(* Logix 5000 Program export EMULATE_TCP_SOCKET; software revision 36.00 *)

TYPE DATATYPE_EMULATION_SOCKET :   // Datatype of FACTORY_IO_SOCKET
STRUCT
   STATUS_CODE : DINT;   // Status code of the socket operation
   CONFIG_SERVER_PORT : STRING_0005;   // Server port number
   CONFIG_SERVER_IP : STRING_0015;   // Server IP address
   CONFIG_MODULE_PATH : STRING;   // Ethernet card path input
   CONFIG_TIMEOUT : DINT;   // Timeout input
   CONFIG_LINGER : DINT;   // Linger input
   CONFIG_QUEUE_SIZE : DINT;
   PARAMS_CREATE_INSTANCE : DINT;   // Instance input
   PARAMS_CREATE : DATATYPE_EMULATION_SOCKET_CREATE;   // Parameters for socket creation
   PARAMS_OPEN : DATATYPE_EMULATION_SOCKET_OPEN;   // Parameters for opening socket
   PARAMS_OPEN_REQUIRED_LENGTH : DINT;
   PARAMS_READ : DATATYPE_EMULATION_SOCKET_READ;   // Parameters for reading from socket
   PARAMS_READ_DESTINATION : DATATYPE_EMULATION_SOCKET_READ_DEST;   // Socket response data
   PARAMS_WRITE : DATATYPE_EMULATION_SOCKET_WRITE;   // Parameters for writing to socket
   PARAMS_WRITE_SIZE_SENT : DINT;   // Size of data sent during write operation
   INPUT_ENABLE_SOCKET : BOOL;   // Enable socket operation
   INPUT_RESET : BOOL;
   READ_LATCH : BOOL;
   READ_QUEUE : STRING_0256[250];
   READ_STRING_ENQUEUE : STRING_0256;
   READ_STRING_ENQUEUE_BUFFER : STRING_3984;
   READ_STRING_ENQUEUE_BUFFER_OLD : STRING_3984;
   READ_STRING_DEQUEUE : STRING_0256;
   READ_TAIL : DINT;
   READ_COUNT : DINT;
   READ_HEAD : DINT;
   WRITE_LATCH : BOOL;
   WRITE_QUEUE : STRING_0256[250];
   WRITE_STRING_ENQUEUE : STRING_0256;
   WRITE_STRING_DEQUEUE : STRING_0256;
   WRITE_HEAD : DINT;
   WRITE_COUNT : DINT;
   WRITE_TAIL : DINT;
   DUMMY_DINT_READ : DINT[5];
   DUMMY_DINT_WRITE : DINT[5];
END_STRUCT
END_TYPE

TYPE DATATYPE_EMULATION_SOCKET_ADDRESS :   // Datatype of FACTORY_IO_SOCKET_ADDRESS
STRUCT
   Family : INT;   // Address Family Must be 2
   Port : INT;   // Port Number
   Addr : SINT[4];   // IP Address
END_STRUCT
END_TYPE

TYPE DATATYPE_EMULATION_SOCKET_CREATE :   // Datatype of FACTORY_IO_SOCKET_CREATE
STRUCT
   Type : DINT;   // 1 - TCP 2- UPD
   Addr : DATATYPE_EMULATION_SOCKET_ADDRESS;   // Socket address information
END_STRUCT
END_TYPE

TYPE DATATYPE_EMULATION_SOCKET_OPEN :   // Datatype of FACTORY_IO_SOCKET_OPEN
STRUCT
   Timeout : DINT;   // Timeout for opening socket
   DestAddr : STRING;   // Destination address
END_STRUCT
END_TYPE

TYPE DATATYPE_EMULATION_SOCKET_READ :   // Datatype of FACTORY_IO_SOCKET_READ
STRUCT
   Timeout : DINT;   // Timeout for reading from socket
   BufLen : DINT;   // Buffer length for read operation
END_STRUCT
END_TYPE

TYPE DATATYPE_EMULATION_SOCKET_READ_DEST :   // Datatype of FACTORY_IO_SOCKET_RESPONSE
STRUCT
   FromAddr : DATATYPE_EMULATION_SOCKET_ADDRESS;   // Source address of the response
   Buffer : STRING_3984;   // Response buffer
END_STRUCT
END_TYPE

TYPE DATATYPE_EMULATION_SOCKET_WRITE :   // Datatype of FACTORY_IO_SOCKET_WRITE
STRUCT
   Timeout : DINT;   // Timeout for writing to socket
   ToAddr : DATATYPE_EMULATION_SOCKET_ADDRESS;   // Destination address for write operation
   Buffer : STRING_3972;   // Write buffer
END_STRUCT
END_TYPE

TYPE STRING_0005 :   // string type
STRUCT
   LEN : DINT;
   DATA : SINT[5];
END_STRUCT
END_TYPE

TYPE STRING_0015 :   // string type
STRUCT
   LEN : DINT;
   DATA : SINT[15];
END_STRUCT
END_TYPE

TYPE STRING_0256 :   // string type
STRUCT
   LEN : DINT;
   DATA : SINT[256];
END_STRUCT
END_TYPE

TYPE STRING_3972 :   // string type
STRUCT
   LEN : DINT;
   DATA : SINT[3972];
END_STRUCT
END_TYPE

TYPE STRING_3984 :   // string type
STRUCT
   LEN : DINT;
   DATA : SINT[3984];
END_STRUCT
END_TYPE

ADD_ON_INSTRUCTION AOI_EMULATION_SOCKET   (* revision 1.0 *)
// AOI to communicate with factory IO
VAR_IN_OUT
   DT_Socket : DATATYPE_EMULATION_SOCKET; {required}   // This tags holds all the data used by the messages
   MSG_Create : MESSAGE; {required}   // Create socket
   MSG_Open : MESSAGE; {required}   // Connect socket to server.
   MSG_Read : MESSAGE; {required}   // Message to tell socket to return any data it has recieved
   MSG_Write : MESSAGE; {required}   // Write socket message
   MSG_Delete : MESSAGE; {required}   // Delete socket
   MSG_Linger : MESSAGE; {required}   // Linger Featuer Message
END_VAR
VAR_OUTPUT
   status_enable : BOOL; {access None, visible}
   status_creating_socket : BOOL; {access None, visible}
   status_connecting : BOOL; {access None, visible}
   status_open : BOOL; {access None, visible}
   status_read : BOOL; {access None, visible}
   status_write : BOOL; {access None, visible}
   status_error : BOOL; {access None, visible}
   status_reading : BOOL; {access None, visible}
   status_writing : BOOL; {access None, visible}
   socket_state : DINT; {access None, visible}
END_VAR
VAR_INPUT
   test_reset_ons : BOOL; {access None, visible}
END_VAR
VAR_OUTPUT
   status_read_queue_not_full : BOOL; {access None, visible}
   max_enque_index : DINT; {access None, visible}
END_VAR
VAR
   State : DINT := 60;   // Current state
   temp : STRING; {access None}
   ons_reset : BOOL; {access None}
   path_string : STRING; {access None}
   read_head : DINT; {access None}
   read_count : DINT; {access None}
   const_port_config : STRING_0015; {access None}
   temp_start_pos : DINT; {access None}
   temp_total_lenght : DINT; {access None}
   temp_index : DINT; {access None}
   const_CRLF : STRING; {access None}
   temp_crlfpos : DINT; {access None}
   temp_string_to_queue : STRING_3984; {access None}
END_VAR

ROUTINE Logic   (* structured text *)
   
   
   if s:fs or (DT_Socket.INPUT_RESET and ons_reset) or test_reset_ons then
   //if  test_reset_ons then ns then
   
   	DT_Socket.CONFIG_QUEUE_SIZE := 200;
   	DT_Socket.READ_HEAD  := 0;
   	DT_Socket.READ_TAIL  := 0;
   	DT_Socket.READ_COUNT := 0;
   	DT_Socket.WRITE_HEAD  := 0;
   	DT_Socket.WRITE_TAIL  := 0;
   	DT_Socket.WRITE_COUNT := 0;
   
   	test_reset_ons := 0;
   	const_port_config := '?PORT=';
   	const_CRLF := '$r$l';
   	max_enque_index := 0;
   
   	path_string := '';
   	CONCAT(path_string, DT_Socket.CONFIG_SERVER_IP, path_string);
   	CONCAT(path_string, const_port_config , path_string);
   	CONCAT(path_string, DT_Socket.CONFIG_SERVER_PORT, path_string);
   	DT_Socket.PARAMS_OPEN.DestAddr := path_string;
   
   	MSG_Create.Path := DT_Socket.CONFIG_MODULE_PATH;
   	MSG_Open.Path 	:= DT_Socket.CONFIG_MODULE_PATH;
   	MSG_Read.Path 	:= DT_Socket.CONFIG_MODULE_PATH;
   	MSG_Write.Path 	:= DT_Socket.CONFIG_MODULE_PATH;
   	MSG_Delete.Path := DT_Socket.CONFIG_MODULE_PATH;
   	MSG_Linger.Path := DT_Socket.CONFIG_MODULE_PATH;
   
   	DT_Socket.PARAMS_OPEN.Timeout 	:= DT_Socket.CONFIG_TIMEOUT;
   	DT_Socket.PARAMS_READ.Timeout 	:= DT_Socket.CONFIG_TIMEOUT;
   	DT_Socket.PARAMS_WRITE.Timeout 	:= DT_Socket.CONFIG_TIMEOUT;
   
   	status_enable			:= 0;
   	status_creating_socket	:= 0;
   	status_connecting		:= 0;
   	status_open				:= 0;
   	status_read				:= 0;
   	status_reading				:= 0;
   	status_write			:= 0;
   	status_writing			:= 0;
   	status_error			:= 0;
   	socket_state := 0;
   
   end_if;
   ons_reset := not DT_Socket.INPUT_RESET;
   
   
   // --- STATE MACHINE FOR TCP CLIENT ---
   CASE socket_state OF
       0: // IDLE / RESET
           socket_state := 10;
       10: // CREATE SOCKET
           //msg_Create.RemoteElement := "";
   		if not MSG_Create.EN then
   			MSG_Create.DN := 0;
   			MSG_Create.ER := 0;
   			MSG(MSG_Create);
   		end_if;
   
           IF MSG_Create.DN THEN
   			MSG_Create.EN := 0;
   			socket_state := 20;
   		end_if;
           IF MSG_Create.ER THEN
   			MSG_Create.EN := 0;
   			socket_state := 100;
   		end_if; // Error
   
   	20: // Lingering
   		MSG_Linger.Instance := DT_Socket.PARAMS_CREATE_INSTANCE;
   		if not MSG_Linger.EN then
   			MSG_Linger.DN := 0;
   			MSG_Linger.ER := 0;
   			MSG(MSG_Linger);
   		end_if;
           IF MSG_Linger.DN THEN
   			MSG_Linger.EN := 0;
   			socket_state := 30;
   		end_if;
           IF MSG_Linger.ER THEN
   			MSG_Linger.EN := 0;
   			socket_state := 100;
   		end_if;
   
       30: // CONNECT TO SERVER
           // Set MyAddress.Addr (Hex), MyAddress.Port, and MyAddress.Family (2)
           MSG_Open.Instance := DT_Socket.PARAMS_CREATE_INSTANCE;
   		MSG_Open.REQ_LEN := DT_Socket.PARAMS_OPEN_REQUIRED_LENGTH;
           if not MSG_Open.EN then
   			MSG_Open.DN := 0;
   			MSG_Open.ER := 0;
   
   			MSG(MSG_Open);
   		end_if;
   
           IF MSG_Open.DN THEN
   			MSG_Open.EN := 0;
   
   			MSG_Read.Instance  := DT_Socket.PARAMS_CREATE_INSTANCE;
   			MSG_Write.Instance := DT_Socket.PARAMS_CREATE_INSTANCE;
   			socket_state := 40;
   		end_if;
           IF MSG_Open.ER THEN
   			MSG_Open.EN := 0;
   			socket_state := 100;
   		end_if;
   
   	40:
   		// Read Logic
   		if not MSG_Read.EN then
   			MSG_Read.DN := 0;
   			MSG_Read.ER := 0;
   			MSG(MSG_Read);
   		end_if;
   
   		if MSG_Read.DN   then
   			MSG_Read.EN := 0;
   			if DT_Socket.PARAMS_READ_DESTINATION.Buffer.LEN > 0 then
   				CONCAT(DT_Socket.READ_STRING_ENQUEUE_BUFFER, DT_Socket.PARAMS_READ_DESTINATION.Buffer, DT_Socket.READ_STRING_ENQUEUE_BUFFER);
   				// here can be added old data not proceeded
   				 DT_Socket.PARAMS_READ_DESTINATION.Buffer.LEN := 0;
   			end_if;
   		end_if;
   
   		IF MSG_Read.ER THEN
   			MSG_Read.EN := 0;
   			socket_state := 100;
   		end_if;
   
   		// Write Logic
   		if DT_Socket.WRITE_LATCH then
   			DT_Socket.WRITE_LATCH := 0;
   			MSG_Write.DN := 0;
   			MSG_Write.ER := 0;
   			COP(DT_Socket.WRITE_STRING_DEQUEUE,DT_Socket.PARAMS_WRITE.Buffer,1);
   			MSG_Write.REQ_LEN := DT_Socket.PARAMS_WRITE.Buffer.LEN + 16;
   			MSG(MSG_Write);
   
   			/*
   			if not MSG_Write.EN  then
   				MSG_Write.DN := 0;
   				MSG_Write.ER := 0;
   
   				COP(DT_Socket.WRITE_STRING_DEQUEUE,DT_Socket.Params_Write.Buffer,1);
   				MSG_Write.REQ_LEN := DT_Socket.Params_Write.Buffer.LEN + 16;
   				MSG(MSG_Write);
   			end_if;
   			*/
   		end_if;
   
   		if MSG_Write.DN  then
   			MSG_Write.EN := 0;
   			MSG_Write.DN := 0;
   			DT_Socket.PARAMS_WRITE.Buffer := '';
   		end_if;
   
   		if MSG_Write.ER then
   			MSG_Write.EN := 0;
   			MSG_Write.ER := 0;
   			socket_state := 100;
   		end_if;
   
       100: // DELETE SOCKET (CLEANUP ON ERROR OR CLOSE)
           MSG_Delete.Instance := DT_Socket.PARAMS_CREATE_INSTANCE;
   		if not MSG_Delete.EN then
   			MSG_Delete.DN := 0;
   			MSG_Delete.ER := 0;
           	MSG(MSG_Delete);
   		end_if;
   
           IF MSG_Delete.DN or MSG_Delete.ER then
   			MSG_Delete.EN := 0;
   			socket_state := 0;
   			//test_reset_ons := 1;
   		end_if;
   END_CASE;
   
   
   //////////////////////////////
   // Write Deque
   IF not DT_Socket.WRITE_LATCH AND MSG_Open.DN and (DT_Socket.WRITE_COUNT > 0) THEN
       CPS(DT_Socket.WRITE_QUEUE[DT_Socket.WRITE_HEAD], DT_Socket.WRITE_STRING_DEQUEUE, 1);
       DT_Socket.WRITE_HEAD := (DT_Socket.WRITE_HEAD + 1) MOD DT_Socket.CONFIG_QUEUE_SIZE;
       DT_Socket.WRITE_COUNT := DT_Socket.WRITE_COUNT - 1;
   	DT_Socket.WRITE_LATCH := 1;
   END_IF;
   
   
   /////////////////////////////
   // Read Enque
   
   temp_start_pos := 1;
   temp_total_lenght := 0;
   temp_crlfpos := 1;
   
   if DT_Socket.READ_STRING_ENQUEUE_BUFFER.LEN > 0 then
   	for temp_index := 0 to 20 do
   
   		if temp_index > max_enque_index then
   			max_enque_index := temp_index ;
   		end_if;
   
   		IF temp_start_pos >= DT_Socket.READ_STRING_ENQUEUE_BUFFER.LEN THEN EXIT; END_IF;
   		FIND(DT_Socket.READ_STRING_ENQUEUE_BUFFER, const_CRLF, temp_start_pos, temp_crlfpos);
   
   		temp_total_lenght := temp_crlfpos - temp_start_pos;
   		 MID(DT_Socket.READ_STRING_ENQUEUE_BUFFER, temp_total_lenght, temp_start_pos, temp_string_to_queue);
   		status_read_queue_not_full := DT_Socket.READ_COUNT < DT_Socket.CONFIG_QUEUE_SIZE;
   
   		IF status_read_queue_not_full THEN
   			CONCAT(temp_string_to_queue, const_CRLF, temp_string_to_queue);
   			CPS( temp_string_to_queue, DT_Socket.READ_QUEUE[DT_Socket.READ_TAIL], 1);
       		DT_Socket.READ_TAIL := (DT_Socket.READ_TAIL + 1) MOD DT_Socket.CONFIG_QUEUE_SIZE;
       		DT_Socket.READ_COUNT := DT_Socket.READ_COUNT + 1;
   		END_IF;
   
   
   		temp_start_pos := temp_crlfpos +2;
   	end_for;
   
   
   
   	DT_Socket.READ_STRING_ENQUEUE_BUFFER := '';
   end_if;
   
   
   /*
   //////////////////////////////
   // Read Deque
   IF not DT_Socket.WRITE_LATCH AND MSG_Open.DN and (read_count > 0) THEN
       CPS(DT_Socket.READ_QUEUE[write_head], DT_Socket.READ_STRING_DEQUEUE, 1);
       read_head := (read_head + 1) MOD DT_Socket.CONFIG_QUEUE_SIZE;
       read_count := read_count - 1;
   	DT_Socket.WRITE_LATCH := 1;
   END_IF;
   */
   
   
   
   
   // HMI
   
   
END_ROUTINE
END_ADD_ON_INSTRUCTION

ADD_ON_INSTRUCTION AOI_EMULATION_SOCKET_DEQUEUE_READ   (* revision 1.0 *)
VAR_IN_OUT
   DT_Socket : DATATYPE_EMULATION_SOCKET; {required}   // This tags holds all the data used by the messages
END_VAR
VAR_OUTPUT
   status_new_messages : BOOL; {access None, visible}
   status_empty : DINT; {access None}
END_VAR
VAR_INPUT
   reset_stats_ons : BOOL; {access None, visible}
END_VAR
VAR_OUTPUT
   counts_good : DINT; {access None, visible}
   counts_bad : DINT; {access None, visible}
END_VAR
VAR
   ons_reset : BOOL; {access None}
   sCrLf : STRING; {access None}
   last_message : STRING_0256; {access None}
   size_message : DINT; {access None}
END_VAR

ROUTINE Logic   (* structured text *)
   
   /* //delete if not used
   
   if s:fs or (DT_Socket.INPUT_RESET and ons_reset)  then
   	DT_Socket.CONFIG_QUEUE_SIZE := 200;
   end_if;
   ons_reset := not DT_Socket.INPUT_RESET;
   */
   
   if reset_stats_ons then
   	reset_stats_ons:= 0;
   	counts_good:= 0;
   	counts_bad:= 0;
   end_if;
   
   status_new_messages := DT_Socket.READ_COUNT > 0;
   
   IF status_new_messages THEN
       CPS(DT_Socket.READ_QUEUE[DT_Socket.READ_HEAD], last_message, 1);
       DT_Socket.READ_HEAD := (DT_Socket.READ_HEAD + 1) MOD DT_Socket.CONFIG_QUEUE_SIZE;
       DT_Socket.READ_COUNT := DT_Socket.READ_COUNT - 1;
   	DT_Socket.READ_LATCH := 1;
   END_IF;
   
   
   // Parse Message
   size_message := 200;
   
   //if (DT_Socket.READ_LATCH and (last_message.DATA[size_message - 2] = 13) and (last_message.DATA[size_message - 1] = 10)) then
   if (last_message.LEN = size_message) then
   	CPS(last_message,DT_Socket.READ_STRING_DEQUEUE, 1);
   
   	counts_good := counts_good +1;
   else
   	counts_bad := counts_bad +1;
   end_if;
   
   
   
   
   
   
   
   
   
END_ROUTINE
END_ADD_ON_INSTRUCTION

ADD_ON_INSTRUCTION AOI_EMULATION_SOCKET_ENQUEUE_SEND   (* revision 1.0 *)
VAR_IN_OUT
   DT_Socket : DATATYPE_EMULATION_SOCKET; {required}   // This tags holds all the data used by the messages
END_VAR
VAR_OUTPUT
   status_full : BOOL; {access None, visible}
   status_empty : DINT; {access None}
END_VAR
VAR
   ons_reset : BOOL; {access None}
   sCrLf : STRING; {access None}
   const_CRLF : STRING; {access None}
   fix_lenght : DINT; {access None}
END_VAR

ROUTINE Logic   (* structured text *)
   
   /* // delete if not used
   if s:fs or (DT_Socket.INPUT_RESET and ons_reset)  then
   	DT_Socket.CONFIG_QUEUE_SIZE := 200;
   end_if;
   ons_reset := not DT_Socket.INPUT_RESET;
   */
   DT_Socket.WRITE_STRING_ENQUEUE.LEN := 198;
   const_CRLF := '$r$l';
   status_full := DT_Socket.WRITE_COUNT > DT_Socket.CONFIG_QUEUE_SIZE;
   
   IF not status_full THEN
   	CONCAT(DT_Socket.WRITE_STRING_ENQUEUE, const_CRLF, DT_Socket.WRITE_STRING_ENQUEUE);
   	CPS( DT_Socket.WRITE_STRING_ENQUEUE, DT_Socket.WRITE_QUEUE[DT_Socket.WRITE_TAIL], 1);
       DT_Socket.WRITE_TAIL := (DT_Socket.WRITE_TAIL + 1) MOD DT_Socket.CONFIG_QUEUE_SIZE;
       DT_Socket.WRITE_COUNT := DT_Socket.WRITE_COUNT + 1;
   END_IF;
   
   
   
   
   
END_ROUTINE
END_ADD_ON_INSTRUCTION

VAR_GLOBAL   (* controller tags *)
   AOI_EMULATION_SOCKET : AOI_EMULATION_SOCKET := (socket_state := 10, status_read_queue_not_full := 1, max_enque_index := 20);
   AOI_EMULATION_SOCKET_DEQUEUE_READ : AOI_EMULATION_SOCKET_DEQUEUE_READ := (counts_good := 37629, counts_bad := 266);
   AOI_EMULATION_SOCKET_ENQUEUE_SEND : AOI_EMULATION_SOCKET_ENQUEUE_SEND := (status_full := 1);
   DT_EMULATION_SOCKET : DATATYPE_EMULATION_SOCKET;
   MSG_EMULATION_CREATE : MESSAGE;
        MessageParameters(MessageType := CIP Generic, RequestedLength := 12, ConnectedFlag := 2, ConnectionPath := 1, 0, ServiceCode := 16#004b, ObjectType := 16#0342, LocalElement := DT_EMULATION_SOCKET.PARAMS_CREATE, DestinationTag := DT_EMULATION_SOCKET.PARAMS_CREATE_INSTANCE)
   MSG_EMULATION_DELETE : MESSAGE;
        MessageParameters(MessageType := CIP Generic, ConnectedFlag := 2, ConnectionPath := 1, 0, ServiceCode := 16#004f, ObjectType := 16#0342, TargetObject := 23064)
   MSG_EMULATION_LINGER : MESSAGE;
        MessageParameters(MessageType := CIP Generic, RequestedLength := 4, ConnectedFlag := 2, ConnectionPath := 1, 0, ServiceCode := 16#0010, ObjectType := 16#0342, TargetObject := 23064, AttributeNumber := 16#000a, LocalElement := DT_EMULATION_SOCKET.CONFIG_LINGER)
   MSG_EMULATION_OPEN : MESSAGE;
        MessageParameters(MessageType := CIP Generic, RequestedLength := 33, ConnectedFlag := 2, ConnectionPath := 1, 0, ServiceCode := 16#004c, ObjectType := 16#0342, TargetObject := 23000, LocalElement := DT_EMULATION_SOCKET.PARAMS_OPEN)
   MSG_EMULATION_READ : MESSAGE;
        MessageParameters(MessageType := CIP Generic, RequestedLength := 8, ConnectedFlag := 2, ConnectionPath := 1, 0, ServiceCode := 16#004d, ObjectType := 16#0342, TargetObject := 21912, LocalElement := DT_EMULATION_SOCKET.PARAMS_READ, DestinationTag := DT_EMULATION_SOCKET.PARAMS_READ_DESTINATION)
   MSG_EMULATION_WRITE : MESSAGE;
        MessageParameters(MessageType := CIP Generic, RequestedLength := 216, ConnectedFlag := 2, ConnectionPath := 1, 0, ServiceCode := 16#004e, ObjectType := 16#0342, TargetObject := 21912, LocalElement := DT_EMULATION_SOCKET.PARAMS_WRITE, DestinationTag := DT_EMULATION_SOCKET.PARAMS_WRITE_SIZE_SENT)
END_VAR

PROGRAM EMULATE_TCP_SOCKET   (* main routine MAIN *)

ROUTINE MAIN   (* structured text *)
   //Call Routines
   JSR(SOCKET_AOI);
   JSR(SOCKET_CONFIGURATION);
   
END_ROUTINE

ROUTINE SOCKET_AOI   (* ladder *)
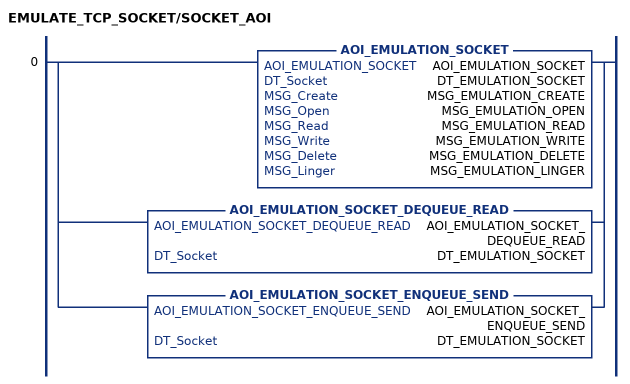
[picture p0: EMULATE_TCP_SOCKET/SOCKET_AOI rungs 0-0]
   0: [AOI_EMULATION_SOCKET(AOI_EMULATION_SOCKET,DT_EMULATION_SOCKET,MSG_EMULATION_CREATE,MSG_EMULATION_OPEN,MSG_EMULATION_READ,MSG_EMULATION_WRITE,MSG_EMULATION_DELETE,MSG_EMULATION_LINGER) ,AOI_EMULATION_SOCKET_DEQUEUE_READ(AOI_EMULATION_SOCKET_DEQUEUE_READ,DT_EMULATION_SOCKET) ,AOI_EMULATION_SOCKET_ENQUEUE_SEND(AOI_EMULATION_SOCKET_ENQUEUE_SEND,DT_EMULATION_SOCKET) ];
END_ROUTINE

ROUTINE SOCKET_CONFIGURATION   (* structured text *)
   
   // SOCKET PARAMETERS
   DT_EMULATION_SOCKET.CONFIG_SERVER_IP 	 		:= '192.168.10.200';
   DT_EMULATION_SOCKET.CONFIG_SERVER_PORT  		:= '42300';
   DT_EMULATION_SOCKET.CONFIG_MODULE_PATH 			:= '$01$00';
   DT_EMULATION_SOCKET.CONFIG_TIMEOUT 				:= 50;  					// Timeout in ms for the Read and Write Service.  Aborts if nothing received in this time
   DT_EMULATION_SOCKET.CONFIG_LINGER 				:= 1;  						// Enable Linger for orderly shutdown of the socket
   DT_EMULATION_SOCKET.PARAMS_OPEN_REQUIRED_LENGTH := 33;
   DT_EMULATION_SOCKET.PARAMS_CREATE.Type 			:= 1; 						//1 For TCP, 2 For UDP
   DT_EMULATION_SOCKET.PARAMS_CREATE.Addr.Family 	:= 2;						//MUST BE 2 Per Rockwell Automation Publication ENET-AT002C-EN-P
   DT_EMULATION_SOCKET.PARAMS_CREATE.Addr.Port 	:= 0; 						//Local Port - Set to 0 to let the EN2T Choose the Local Port
   DT_EMULATION_SOCKET.PARAMS_READ.BufLen 			:= 484;						// 484 bytes for Standard Connection, 3984 Bytes for Large connection
   DT_EMULATION_SOCKET.PARAMS_WRITE.ToAddr.Family 	:= 2;
   
   
END_ROUTINE
END_PROGRAM
